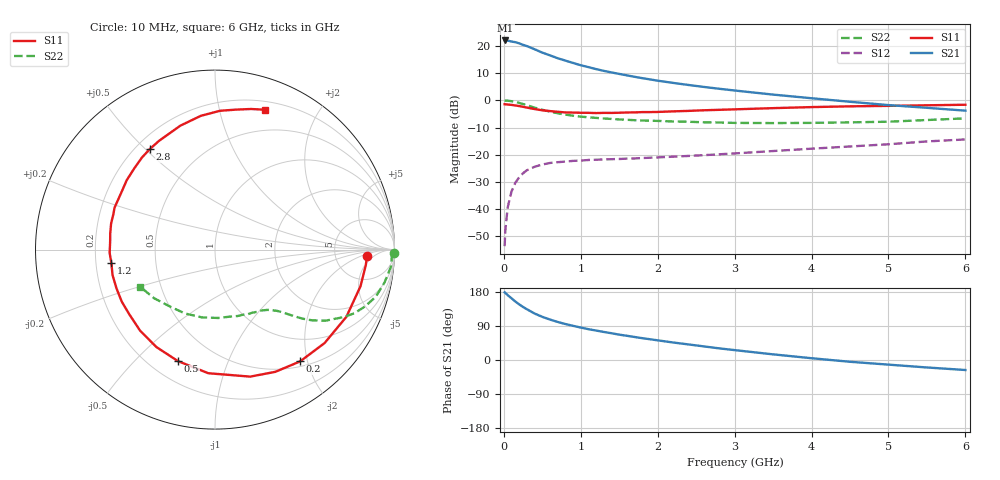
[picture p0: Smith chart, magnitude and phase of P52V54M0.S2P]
! SIEMENS Small Signal Semiconductors
! BFP183
! Si NPN RF Bipolar Junction Transistor in SOT143
! VCE = 2.5 V  IC = 4 mA
! Common Emitter S-Parameters:  March  1996
# GHz  S  MA  R  50
!  f  S11  S21  S12  S22
! GHz  MAG  ANG  MAG  ANG  MAG  ANG  MAG  ANG
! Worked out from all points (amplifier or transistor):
!   36 points, 10 MHz to 6 GHz, reference 50 ohm
!   highest |S21| = 22.0 dB at 20 MHz (marker M1)
!   |S21| within 3 dB of that: start of sweep to 380.1 MHz
!   unconditionally stable (mu >= 1): 1.683 GHz to 5.725 GHz
!   at 250 MHz: K = 0.18, MSG = 23.6 dB, |S12| = -26.8 dB
!   at 1.4 GHz: K = 0.88, MSG = 15.9 dB, |S12| = -21.6 dB
!   at 6 GHz: K = 0.96, MSG = 5.3 dB, |S12| = -14.4 dB
!   S11 on the Smith chart (normalised r, x): 10 MHz: 11, -3; 200 MHz: 0.58, -1.88; 500 MHz: 0.31, -0.67; 1.2 GHz: 0.27, -0.06; 2.8 GHz: 0.26, +0.52; 6 GHz: 0.28, +1.38
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0.01  0.8468 -2.6  12.39 178.5  0.0021 82.4  0.9952 -1.2
0.02  0.845 -5.7  12.53 177.0  0.0042 88.5  0.9863 -2.2
0.05  0.8361 -14.1  12.46 171.1  0.0108 83.9  0.9846 -5.6
0.15  0.8025 -40.4  11.64 154.3  0.0307 68.8  0.9337 -16.3
0.2  0.7829 -52.7  11.09 146.7  0.0387 63.2  0.8945 -20.7
0.25  0.7595 -63.7  10.4 139.9  0.0458 57.8  0.8541 -24.5
0.3  0.7344 -74.5  9.867 133.9  0.052 53.4  0.8109 -27.6
0.4  0.6898 -93.1  8.636 122.6  0.0602 45.8  0.7329 -32.7
0.5  0.6547 -108.4  7.488 113.9  0.0662 40.0  0.6689 -36.1
0.6  0.6334 -121.1  6.67 106.7  0.0707 36.1  0.6186 -38.4
0.7  0.6148 -132.8  5.907 100.4  0.073 33.0  0.5779 -40.0
0.8  0.5984 -142.8  5.348 94.9  0.075 30.5  0.5458 -41.4
1.1  0.5882 -166.1  4.056 81.3  0.0802 26.7  0.4865 -44.6
1.2  0.5823 -172.5  3.731 77.7  0.081 25.7  0.4747 -45.7
1.5  0.5907 171.2  3.047 66.9  0.0836 25.3  0.4448 -49.0
1.7  0.5991 161.3  2.696 60.7  0.0857 25.4  0.4305 -51.8
2.2  0.6257 141.8  2.085 46.2  0.0922 26.3  0.4082 -59.5
2.8  0.6679 122.8  1.626 30.7  0.1019 27.4  0.391 -71.2
3.5  0.717 105.6  1.271 14.9  0.117 28.2  0.3814 -87.2
4.5  0.774 87.9  0.938 -4.7  0.1419 25.9  0.3932 -115.1
5.5  0.8088 75.6  0.727 -19.7  0.1757 22.0  0.4342 -141.4
6  0.8277 70.3  0.645 -26.4  0.1911 18.1  0.4656 -153.6
